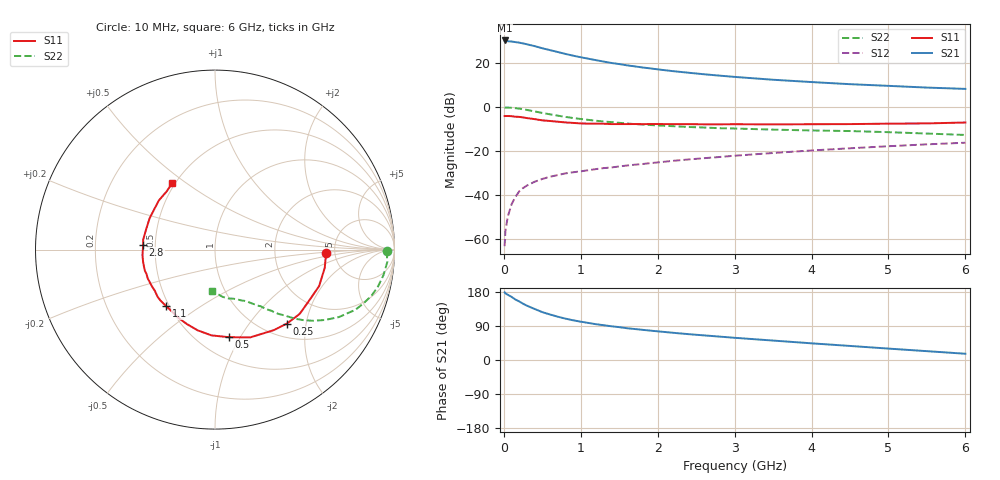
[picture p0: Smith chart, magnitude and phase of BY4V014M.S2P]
! SIEMENS Small Signal Semiconductors
! BFY420
! Si NPN RF SIEGET Grounded Emitter Transistor in MICRO-X
! VCE = 4 V  IC = 14 mA
! Common Emitter S-Parameters:  October  1996
# GHz  S  MA  R  50
!  f  S11  S21  S12  S22
! GHz  MAG  ANG  MAG  ANG  MAG  ANG  MAG  ANG
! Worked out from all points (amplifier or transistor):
!   36 points, 10 MHz to 6 GHz, reference 50 ohm
!   highest |S21| = 30.1 dB at 10 MHz (marker M1)
!   |S21| within 3 dB of that: start of sweep to 445 MHz
!   unconditionally stable (mu >= 1): start of sweep to 18.53 MHz; 2.296 GHz to end of sweep
!   at 250 MHz: K = 0.28, MSG = 32.7 dB, |S12| = -36.8 dB
!   at 1.4 GHz: K = 0.84, MSG = 23.7 dB, |S12| = -27.5 dB
!   at 6 GHz: K = 1.07, MAG = 10.6 dB, |S12| = -16.2 dB
!   S11 on the Smith chart (normalised r, x): 10 MHz: 4.20, -0.28; 250 MHz: 1.27, -1.56; 500 MHz: 0.69, -0.89; 1.1 GHz: 0.48, -0.37; 2.8 GHz: 0.43, +0.03; 6 GHz: 0.48, +0.45
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0.01  0.617 -1.9  31.82 178.5  0.0007 33.5  0.9606 -0.5
0.02  0.6184 -3.9  31.62 175.9  0.0015 47.8  0.9575 -1.4
0.05  0.6198 -9.4  30.61 172.3  0.0032 71.1  0.9625 -4.1
0.1  0.6147 -19.3  30.08 166.6  0.0062 76.1  0.9499 -8.5
0.15  0.5971 -28.0  29.23 159.6  0.0091 71.8  0.9315 -12.7
0.2  0.5924 -37.2  28.39 154.5  0.0122 70.5  0.9094 -16.4
0.25  0.5749 -45.8  27.24 148.5  0.0145 67.7  0.8792 -20.0
0.3  0.5559 -53.8  26.07 143.3  0.0165 65.9  0.8511 -23.2
0.4  0.527 -68.2  23.68 134.7  0.0201 62.1  0.787 -28.5
0.5  0.4937 -81.2  21.2 126.3  0.0233 59.3  0.7278 -32.6
0.7  0.4601 -102.1  17.45 114.3  0.0285 56.6  0.632 -38.5
0.8  0.4434 -110.7  15.78 109.2  0.0311 55.0  0.5914 -40.7
0.9  0.4324 -117.5  14.39 104.8  0.033 54.5  0.5585 -42.2
1.1  0.4162 -130.9  12.27 97.8  0.0368 54.7  0.506 -45.2
1.3  0.4138 -140.8  10.55 91.7  0.041 54.4  0.4655 -47.2
1.6  0.4064 -153.3  8.71 83.9  0.0469 54.7  0.4197 -50.3
2.2  0.4062 -170.8  6.418 71.8  0.0599 53.9  0.3646 -55.5
2.8  0.4012 176.0  5.093 61.8  0.073 52.3  0.3282 -60.3
3.5  0.3999 163.2  4.103 51.3  0.0901 48.9  0.3046 -65.8
4.5  0.4064 146.4  3.257 37.1  0.1152 42.2  0.2829 -74.3
5.5  0.4213 129.8  2.727 23.3  0.1414 34.2  0.2483 -86.5
6  0.4417 122.5  2.548 16.5  0.154 29.7  0.2306 -94.3
